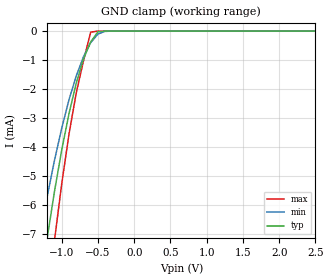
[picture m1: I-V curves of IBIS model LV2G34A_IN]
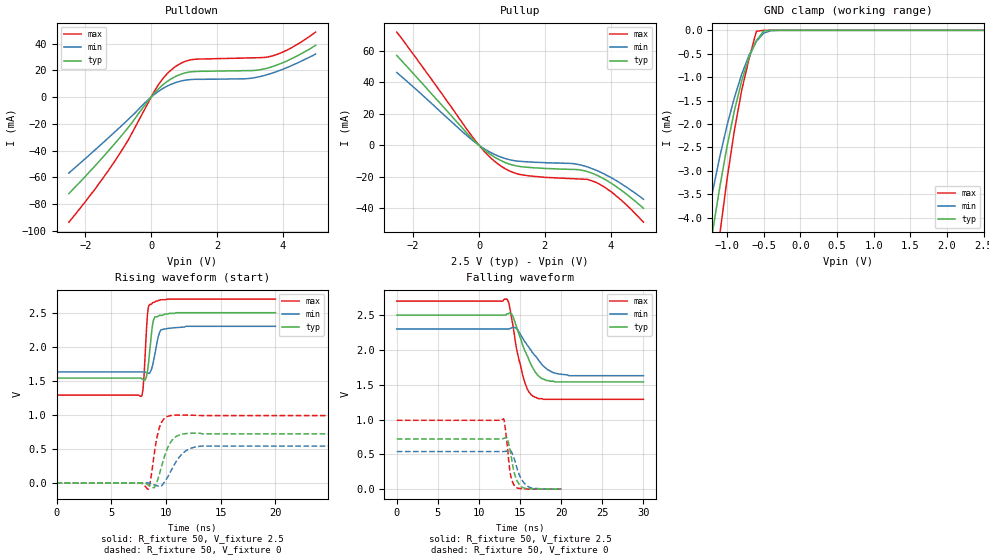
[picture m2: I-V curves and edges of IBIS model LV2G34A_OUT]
|/_/_/_/_/_/_/_/_/_/_/_/_/_/_/_/_/_/_/_/_/_/_/_/_/_/_/_/_/_/_/_/_/_/_/_/_/_/
|   Renesas Electronics Corp.
|   Multi Purpose Semiconductor Digital IC Design Group
|   IBIS Model of HD74LV2G34A
|   2.5V Triple Noninverters,  SSOP-8(8pin) Package
|   History
|   V1.0   April   1, 2003   : First release.
|/_/_/_/_/_/_/_/_/_/_/_/_/_/_/_/_/_/_/_/_/_/_/_/_/_/_/_/_/_/_/_/_/_/_/_/_/_/
[IBIS Ver]   2.1
[Comment Char]  |_char
[File name]   l2g34s2.ibs
[File Rev]   1.1
[Date]   April 1, 2003
[Source]   Data created from SPICE simulations at
|   Renesas Electronics Corp.
[Notes]   RLC value of the Package is determined by assuming typical
|   conditions.
[Disclaimer]   This information is for modeling purposes only, and is not
|   guaranteed.
[Copyright]   (C) Copyright 2003, Renesas Electronics Corp.,
|   All Rights Reserved.
|   Component  HD74LV2G34A
[Component]   HD74LV2G34A
[Manufacturer]  Renesas Electronics Corp.
[Package]
|   typ   min   max
R_pkg   0.099   0.095   0.102
L_pkg   1.740nH   1.680nH   1.790nH
C_pkg   0.140pF   0.140pF   0.150pF
[Pin]   signal_name   model_name   R_pin   L_pin   C_pin
1   1A   LV2G34A_IN   0.102   1.780nH   0.140pF
2   3Y   LV2G34A_OUT   0.097   1.710nH   0.150pF
3   2A   LV2G34A_IN   0.095   1.680nH   0.150pF
4   GND   GND   0.102   1.790nH   0.140pF
5   2Y   LV2G34A_OUT   0.101   1.790nH   0.140pF
6   3A   LV2G34A_IN   0.097   1.710nH   0.150pF
7   1Y   LV2G34A_OUT   0.097   1.710nH   0.150pF
8   VCC   POWER   0.102   1.790nH   0.140pF
| Models and submodels in the file (2): LV2G34A_IN (Input), LV2G34A_OUT (Output)
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|   Model  LV2G34A_IN
[Model]   LV2G34A_IN
Model_type  Input
Vinl = 0.75V
Vinh = 1.75V
| variable   typ   min   max
C_comp   2.35pF   2.25pF   2.45pF
| variable   typ   min   max
[Temperature range]   25   85   -40
| variable   typ   min   max
[Voltage range]   2.5V   2.3V   2.7V
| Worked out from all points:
|   GND clamp passes 1 mA (typ) near -0.70 V on its own axis
[GND Clamp]
|   Voltage   I(typ)   I(min)   I(max)
-2.5V     -38.3mA    -30.7mA    -49.7mA
-1.3V     -8.88mA    -7.07mA    -11.7mA
-1.2V     -7.13mA    -5.7mA     -9.39mA
-1.1V     -5.53mA    -4.46mA    -7.22mA
-1V       -4.1mA     -3.35mA    -5.27mA
-900mV    -2.85mA    -2.37mA    -3.56mA
-800mV    -1.8mA     -1.55mA    -2.14mA
-700mV    -962uA     -887uA     -1.03mA
-600mV    -372uA     -399uA     -36.9uA
-500mV    -22uA      -101uA     -445nA
-400mV    -433nA     -10.3uA    -2.54nA
2.5V      5.09pA     27.7pA     5pA
|   Model  LV2G34A_OUT
[Model]   LV2G34A_OUT
Model_type  Output
Polarity   Inverting
Vmeas = 1.25V
| variable   typ   min   max
C_comp   6.35pF   6.25pF   6.45pF
| variable   typ   min   max
[Temperature range]   25   85   -40
| variable   typ   min   max
[Voltage range]   2.5V   2.3V   2.7V
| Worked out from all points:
|   slope of the pulldown table from 0 to 0.375 V, typ, clamps not added: 39.2 ohm
|   slope of the pullup table from 0 to 0.375 V, typ, clamps not added: 60.8 ohm
|   GND clamp passes 1 mA (typ) near -0.78 V on its own axis
|   rising waveform, R_fixture 50, V_fixture 2.5: 20-80 % time 380ps typ, 502ps min, 288ps max; typ from 1.54 V to 2.5 V
|   rising waveform, R_fixture 50, V_fixture 0: 20-80 % time 922ps typ, 1.29ns min, 629ps max; typ from 0 V to 0.721 V
|   falling waveform, R_fixture 50, V_fixture 2.5: 20-80 % time 1.96ns typ, 2.54ns min, 1.45ns max; typ from 2.5 V to 1.54 V
|   falling waveform, R_fixture 50, V_fixture 0: 20-80 % time 798ps typ, 1.07ns min, 579ps max; typ from 0.721 V to 0 V
[Pullup]
|   Voltage   I(typ)   I(min)   I(max)
-2.5V     56.9mA     46.1mA     71.7mA
-200mV    4.01mA     3.18mA     5.31mA
200mV     -3.53mA    -2.75mA    -4.76mA
500mV     -7.83mA    -6.06mA    -10.6mA
900mV     -11.7mA    -8.98mA    -16mA
1.2V      -13.3mA    -10.1mA    -18.3mA
2.9V      -15.3mA    -11.7mA    -21.2mA
3.3V      -16.7mA    -13.7mA    -21.6mA
3.5V      -18.2mA    -15.3mA    -23mA
4.1V      -25.1mA    -21.5mA    -30.8mA
4.5V      -31.2mA    -26.7mA    -38.1mA
5V        -39.9mA    -34.2mA    -48.7mA
[Pulldown]
|   Voltage   I(typ)   I(min)   I(max)
-2.5V     -72mA      -56.7mA    -93.4mA
-1.7V     -51.2mA    -39.3mA    -68.5mA
-1.1V     -34.6mA    -25.9mA    -47.7mA
-700mV    -22.8mA    -16.8mA    -32.2mA
200mV     5.59mA     3.93mA     8.44mA
700mV     14.9mA     10.5mA     22.1mA
1V        17.9mA     12.5mA     26.4mA
1.3V      19.1mA     13.3mA     28.2mA
2.9V      19.8mA     13.8mA     29.3mA
3.7V      22.9mA     18.1mA     30.9mA
4.3V      29.1mA     23.9mA     37.3mA
5V        38.7mA     32.2mA     48.6mA
[GND Clamp]
|   Voltage   I(typ)   I(min)   I(max)
-2.5V     -23.4mA    -18.8mA    -30.3mA
-1.3V     -5.4mA     -4.31mA    -7.13mA
-1.2V     -4.33mA    -3.47mA    -5.69mA
-1.1V     -3.36mA    -2.71mA    -4.37mA
-1V       -2.48mA    -2.03mA    -3.18mA
-900mV    -1.72mA    -1.44mA    -2.14mA
-800mV    -1.08mA    -936uA     -1.28mA
-700mV    -575uA     -533uA     -610uA
-600mV    -219uA     -237uA     -20.5uA
-500mV    -12.9uA    -58.6uA    -245nA
-400mV    -248nA     -6.13uA    -1.4nA
2.5V      2.62pA     30.9pA     2.5pA
[Ramp]
| variable   typ   min   max
dV/dt_r   0.432/920.2p   0.324/1.288n   0.593/628.8p
dV/dt_f   0.578/1.959n   0.400/2.545n   0.847/1.439n
R_load = 50ohms
[Rising Waveform]
R_fixture = 50
V_fixture = 2.5
V_fixture_min = 2.3
V_fixture_max = 2.7
C_fixture = 0p
|   Time   V(typ)   V(min)   V(max)
0s        1.54V      1.63V      1.29V
7.8ns     1.53V      1.63V      1.28V
7.9ns     1.52V      1.63V      1.37V
8ns       1.51V      1.63V      1.58V
8.3ns     1.63V      1.62V      2.46V
8.4ns     1.75V      1.61V      2.59V
8.8ns     2.35V      1.74V      2.65V
9.3ns     2.45V      2.15V      2.68V
9.6ns     2.46V      2.25V      2.69V
20ns      2.5V       2.3V       2.7V
[Rising Waveform]
R_fixture = 50
V_fixture = 0
C_fixture = 0p
|   Time   V(typ)   V(min)   V(max)
0s        496pV      604nV      132pV
7.7ns     496pV      604nV      132pV
8.4ns     -30.7mV    471uV      -91mV
8.9ns     -71.7mV    -27.4mV    392mV
9.4ns     131mV      -50.4mV    812mV
9.8ns     357mV      331uV      938mV
10.4ns    592mV      160mV      989mV
11.6ns    720mV      445mV      996mV
13.2ns    728mV      541mV      990mV
35ns      721mV      541mV      989mV
[Falling Waveform]
R_fixture = 50
V_fixture = 2.5
V_fixture_min = 2.3
V_fixture_max = 2.7
C_fixture = 0p
|   Time   V(typ)   V(min)   V(max)
0s        2.5V       2.3V       2.7V
13.4ns    2.52V      2.3V       2.73V
14ns      2.51V      2.32V      2.43V
14.6ns    2.32V      2.3V       1.99V
15.3ns    2.07V      2.17V      1.64V
15.9ns    1.91V      2.06V      1.43V
16.6ns    1.73V      1.95V      1.33V
17.6ns    1.59V      1.8V       1.3V
19.4ns    1.54V      1.66V      1.29V
30ns      1.54V      1.63V      1.29V
[Falling Waveform]
R_fixture = 50
V_fixture = 0
C_fixture = 0p
|   Time   V(typ)   V(min)   V(max)
0s        721mV      540mV      989mV
13ns      728mV      540mV      1.01V
13.1ns    733mV      541mV      957mV
13.4ns    738mV      548mV      665mV
13.8ns    542mV      557mV      226mV
14.1ns    338mV      493mV      96.4mV
14.4ns    187mV      393mV      35.3mV
15ns      52.8mV     178mV      9.5mV
16ns      8.26mV     35.5mV     1.27mV
20ns      -19uV      -44.4uV    -4.37uV
